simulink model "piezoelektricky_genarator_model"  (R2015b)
settings: Solver=VariableStepAuto  StartTime=0.0  StopTime=t  FixedStep=1e-4  RelTol=1e-3
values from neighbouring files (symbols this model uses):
  b = 2*b_p*m*ome    (= 415.611533333)    [P_016_80_parametry.m]    (also in parametry_magneto.m = 2*b_p*m_t*ome)
  b_amp = 2*0.02*m_amp*ome_amp    (= 3.90920092413)    [piezoelektricky_genarator_parametry.m]    (also in parametry_magneto.m = 29.2857142857)
  C = 1.7e-6    (= 1.7e-06)    [piezoelektricky_genarator_parametry.m]    (also in P_016_80_parametry.m = 1.3e-06)
  d33 = 6.5e-10    [P_016_80_parametry.m]    (also in parametry_magneto.m = 2e-09)
  delta_x = 4e-4    (= 0.0004)    [piezoelektricky_genarator_parametry.m]    (also in parametry_magneto.m)
  k = 56e+6    (= 56000000)    [P_016_80_parametry.m]    (also in parametry_magneto.m = 1005309649.15)
  k_a = 12.3e7    (= 123000000)    [piezoelektricky_genarator_parametry.m]
  k_amp = F_in/delta_x    (= 6821500)    [piezoelektricky_genarator_parametry.m]    (also in parametry_magneto.m)
  m = m_eff+m_amp    [piezoelektricky_genarator_parametry.m]    (also in P_016_80_parametry.m = 0.1804; parametry_magneto.m = 2.02300536849)
  n = floor(C*h/(8.854188e-12*e33_e0*A))    [P_016_80_parametry.m]
  R = 45000    [piezoelektricky_genarator_parametry.m]

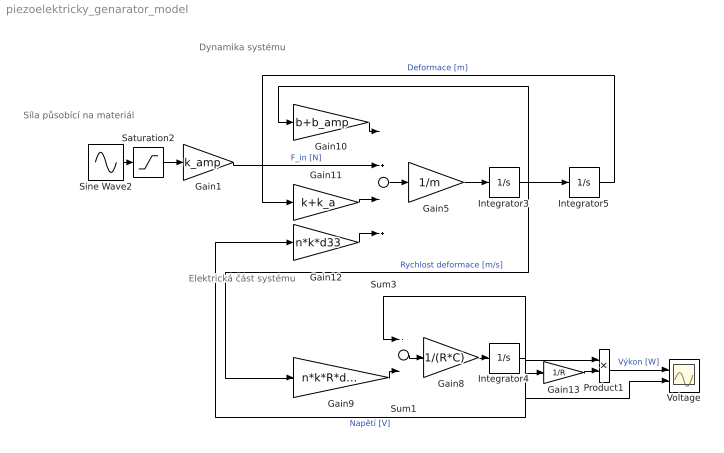
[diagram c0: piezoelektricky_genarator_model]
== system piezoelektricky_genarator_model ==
  note: Elektrická část systému
  note: Dynamika systému
  note: Síla působící na materiál
  Gain1 : Gain  Gain=k_amp
  Gain10 : Gain  Gain=b+b_amp
  Gain11 : Gain  Gain=k+k_a
  Gain12 : Gain  Gain=n*k*d33
  Gain13 : Gain  Gain=1/R
  Gain5 : Gain  Gain=1/m
  Gain8 : Gain  Gain=1/(R*C)
  Gain9 : Gain  Gain=n*k*R*d33
  Integrator3 : Integrator
  Integrator4 : Integrator
  Integrator5 : Integrator
  Product1 : Product
  Saturation2 : Saturate  UpperLimit=delta_x  LowerLimit=0
  Sine Wave2 : Sin  Amplitude=2*delta_x  Frequency=2*pi*2  SampleTime=0
  Sum1 : Sum  Inputs=--
  Sum3 : Sum  Inputs=-+-+
  Voltage : Scope  NumInputPorts=2
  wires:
  Gain5/1 -> Integrator3/1
  Gain8/1 -> Integrator4/1
  Sum1/1 -> Gain8/1
  Integrator4/1 -> Gain13/1, Gain12/1, Voltage/2, Product1/1, Sum1/1  "Napětí [V]"
  Gain9/1 -> Sum1/2
  Sum3/1 -> Gain5/1
  Gain10/1 -> Sum3/1
  Integrator3/1 -> Integrator5/1, Gain10/1, Gain9/1  "Rychlost deformace [m/s]"
  Gain11/1 -> Sum3/3
  Integrator5/1 -> Gain11/1  "Deformace [m]"
  Gain12/1 -> Sum3/4
  Gain13/1 -> Product1/2
  Product1/1 -> Voltage/1  "Výkon [W]"
  Sine Wave2/1 -> Saturation2/1
  Gain1/1 -> Sum3/2  "F_in [N]"
  Saturation2/1 -> Gain1/1
